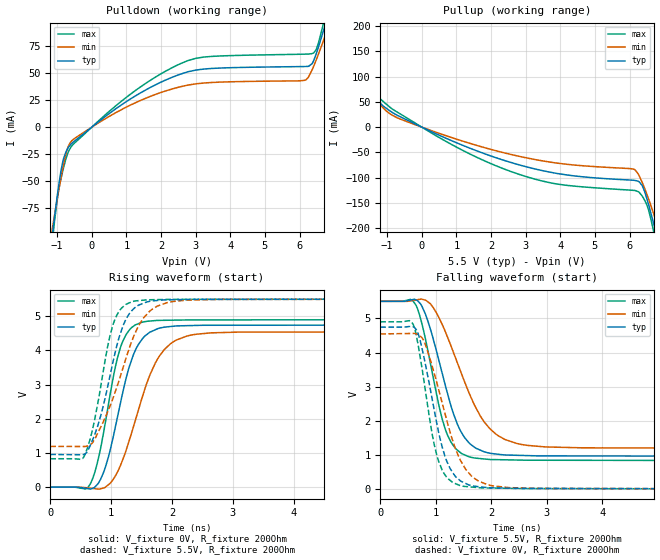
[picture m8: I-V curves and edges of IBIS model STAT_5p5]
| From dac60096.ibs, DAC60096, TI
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|   Model
[Model]   STAT_5p5
Model_type   Output
Polarity   Non-Inverting
Vmeas = 2.75
Vref = 0
Cref = 1pF
Rref = 100000
|   typ   min   max
C_comp   12.144pF   11.345pF   12.754pF
[Voltage Range]   5.5   5.499   5.501
[Temperature Range]   27   105   -40
[Pullup Reference]   5.5   5.499   5.501
[Pulldown Reference]   0   0   0
[Power Clamp Reference]   5.5   5.499   5.501
[GND Clamp Reference]   0   0   0
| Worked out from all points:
|   slope of the pulldown table from 0 to 0.825 V, typ, clamps not added: 41.5 ohm
|   slope of the pullup table from 0 to 0.825 V, typ, clamps not added: 32 ohm
|   falling waveform, V_fixture 5.5V, R_fixture 200Ohm: 20-80 % time 480ps typ, 672ps min, 379ps max; typ from 5.5 V to 0.955 V
|   rising waveform, V_fixture 0V, R_fixture 200Ohm: 20-80 % time 386ps typ, 514ps min, 318ps max; typ from 0 V to 4.74 V
|   rising waveform, V_fixture 5.5V, R_fixture 200Ohm: 20-80 % time 379ps typ, 523ps min, 298ps max; typ from 0.955 V to 5.5 V
|   falling waveform, V_fixture 0V, R_fixture 200Ohm: 20-80 % time 372ps typ, 495ps min, 308ps max; typ from 4.74 V to 0.001 V
[Pulldown]
|   Voltage   I(typ)   I(min)   I(max)
-5.5V     -1.394A    -1.139A    -1.672A
-1.111V   -91.71mA   -88.14mA   -97.07mA
-979mV    -59.16mA   -62.61mA   -62.22mA
-847mV    -33.24mA   -39.43mA   -41.56mA
-599.5mV  -15.7mA    -13.24mA   -18.2mA
1.216V    28.04mA    21.91mA    32.84mA
2.783V    51.25mA    38.92mA    61.63mA
6.165V    56.09mA    43.4mA     67.52mA
6.364V    58.71mA    52.96mA    68.02mA
6.726V    92.94mA    83.05mA    100.4mA
6.875V    109.3mA    96.26mA    120.9mA
11V       618.7mA    512.3mA    755.9mA
[Pullup]
|   Voltage   I(typ)   I(min)   I(max)
-5.5V     534.6mA    445.4mA    662.9mA
-4.345V   400.6mA    331.2mA    493.9mA
-2.497V   187.4mA    159.8mA    224.6mA
-2.365V   172.3mA    147.7mA    205.6mA
-1.375V   62.55mA    58.77mA    68.98mA
-847mV    28.77mA    23.33mA    35.57mA
2.783V    -74.14mA   -57.34mA   -92.85mA
6.116V    -105.2mA   -83.16mA   -125.2mA
6.364V    -115.4mA   -108.9mA   -136.1mA
6.71V     -194.3mA   -174mA     -211.1mA
6.875V    -239.2mA   -208.6mA   -266.7mA
11V       -1.473A    -1.207A    -1.76A
[Ramp]
R_load = 200
|   typ   min   max
dV/dt_r   2.8466/3.85087e-10   2.72691/5.14417e-10   2.93993/3.16709e-10
dV/dt_f   2.72679/4.79819e-10   2.58413/6.72206e-10   2.80225/3.78797e-10
[Falling Waveform]
V_fixture = 5.5V
V_fixture_min = 5.499V
V_fixture_max = 5.501V
R_fixture = 200Ohm
C_fixture = 0F
|   Time   V(typ)   V(min)   V(max)
0s        5.5V       5.499V     5.501V
545.5ps   5.537V     5.514V     5.555V
734ps     5.404V     5.565V     4.943V
912.1ps   4.637V     5.41V      3.613V
1.171ns   3.045V     4.615V     1.758V
1.39ns    1.903V     3.698V     1.142V
1.595ns   1.364V     2.837V     951.1mV
1.974ns   1.053V     1.772V     868.9mV
2.644ns   983.5mV    1.283V     847.6mV
10ns      955.3mV    1.192V     830.6mV
[Rising Waveform]
V_fixture = 0V
V_fixture_min = 0V
V_fixture_max = 0V
R_fixture = 200Ohm
C_fixture = 0F
|   Time   V(typ)   V(min)   V(max)
0s        -22.47nV   -106.8nV   -63.57nV
615.1ps   -43.78mV   -22.36mV   -15.21mV
798.6ps   137.3mV    -58.25mV   900.9mV
954.1ps   872.6mV    68.13mV    2.394V
1.15ns    2.431V     618.3mV    4.066V
1.297ns   3.513V     1.359V     4.589V
1.506ns   4.318V     2.596V     4.822V
1.879ns   4.68V      4.031V     4.88V
2.386ns   4.729V     4.469V     4.892V
10ns      4.744V     4.545V     4.9V
[Rising Waveform]
V_fixture = 5.5V
V_fixture_min = 5.499V
V_fixture_max = 5.501V
R_fixture = 200Ohm
C_fixture = 0F
|   Time   V(typ)   V(min)   V(max)
0s        955mV      1.191V     830.5mV
556.4ps   962mV      1.188V     897.8mV
659.8ps   1.23V      1.246V     1.436V
782.2ps   1.804V     1.585V     2.461V
1.02ns    3.571V     2.543V     4.681V
1.193ns   4.706V     3.476V     5.27V
1.339ns   5.158V     4.264V     5.422V
1.666ns   5.444V     5.192V     5.482V
2.248ns   5.49V      5.469V     5.493V
10ns      5.5V       5.499V     5.501V
[Falling Waveform]
|Gnd
V_fixture = 0V
V_fixture_min = 0V
V_fixture_max = 0V
R_fixture = 200Ohm
C_fixture = 0F
|   Time   V(typ)   V(min)   V(max)
0s        4.744V     4.545V     4.9V
525.8ps   4.763V     4.558V     4.934V
659ps     4.644V     4.543V     4.424V
796.8ps   3.789V     4.296V     3.062V
1.02ns    1.915V     3.114V     987mV
1.193ns   836.8mV    2.045V     356.3mV
1.43ns    262.7mV    892.1mV    110.1mV
1.76ns    75.87mV    245.3mV    46.66mV
2.315ns   29.35mV    45.85mV    25.24mV
10ns      503.2uV    1.443mV    111.3uV
